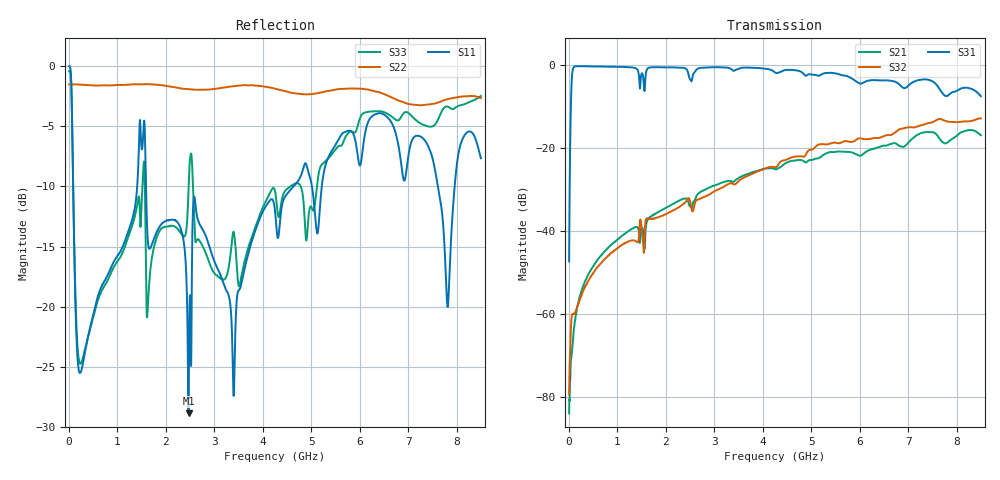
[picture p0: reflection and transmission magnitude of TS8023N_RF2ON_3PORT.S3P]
!Agilent Technologies,E5071C,MY46522130,B.12.04
!Date: Thu Jul 17 20:32:42 2025
!Data & Calibration Information:
!Freq	S11:SOLT3(ON)	S13:SOLT3(ON)	S14:SOLT3(ON)
!	S31:SOLT3(ON)	S33:SOLT3(ON)	S34:SOLT3(ON)
!	S41:SOLT3(ON)	S43:SOLT3(ON)	S44:SOLT3(ON)
!PortZ  Port1:50+j0  Port3:50+j0  Port4:50+j0
!Above PortZ is port z conversion or system Z0 setting when saving the data.
!When reading, reference impedance value at option line is always used.
# Hz S dB R 50
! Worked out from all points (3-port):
!   1601 points, 10 MHz to 8.5 GHz, reference 50 ohm
!   strongest paths, dB at 10 MHz, 2.132 GHz, 4.255 GHz, 6.378 GHz, 8.5 GHz:
!     S31: -47.3, -0.5, -1.7, -3.6, -7.4
!     S32: -79.4, -35.1, -24.6, -17.5, -12.8
!     S21: -84.0, -33.6, -25.1, -19.8, -16.8
!   lowest |S11| = -28.9 dB at 2.472 GHz (marker M1), VSWR 1.07, Z = 50.7 - j3.57 ohm
!   |S11| at or under -10 dB: 92.97 MHz to 1.413 GHz (1.32 GHz wide, 175 % of centre); 1.595 GHz to 4.636 GHz (3.041 GHz wide, 97.6 % of centre); 7.614 GHz to 7.959 GHz (345.3 MHz wide, 4.43 % of centre)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
1e7  0.00 163.0  -84.50 89.5  -47.36 -111.1
     -84.01 79.7  -1.52 179.8  -79.41 -109.2
     -47.31 -110.6  -79.43 -111.5  -0.42 162.0
6.836875e7  -3.80 42.9  -69.42 -74.2  -2.70 128.9
            -69.32 -74.2  -1.51 179.1  -60.24 137.2
            -2.71 128.8  -60.29 136.2  -3.84 35.4
1.267375e8  -17.56 -19.3  -61.94 169.8  -0.25 60.6
            -61.99 168.3  -1.51 178.4  -59.87 98.6
            -0.25 60.6  -60.00 100.3  -16.88 -35.9
4.238875e8  -22.10 -64.3  -50.08 112.0  -0.19 9.1
            -50.07 112.2  -1.57 174.4  -51.68 94.7
            -0.19 9.2  -51.68 94.4  -22.15 -87.6
1.522281e9  -6.65 -107.0  -39.21 94.0  -2.04 -28.2
            -39.23 93.9  -1.50 158.7  -40.78 83.4
            -2.04 -28.2  -40.76 83.3  -9.94 -145.2
2.4721e9  -28.86 -77.5  -33.23 82.3  -2.16 -54.7
          -33.16 82.5  -1.91 145.9  -32.03 86.0
          -2.16 -54.7  -32.07 86.0  -10.19 -125.0
4.255e9  -12.02 154.4  -25.17 66.8  -1.69 -83.5
         -25.06 67.2  -1.87 125.0  -24.46 73.9
         -1.70 -83.6  -24.58 73.5  -10.38 -167.3
6.478319e9  -3.96 142.5  -19.46 33.4  -3.62 -122.3
            -19.40 33.3  -2.27 97.0  -17.06 22.9
            -3.58 -122.3  -17.14 23.4  -3.78 154.3
7.815494e9  -20.02 131.9  -18.92 10.5  -7.31 -144.0
            -18.56 8.4  -2.74 56.1  -13.40 -14.8
            -7.30 -144.0  -13.56 -12.0  -3.36 116.6
8.5e9  -7.65 100.1  -16.77 -6.8  -7.45 -159.3
       -16.84 -5.3  -2.65 62.4  -12.74 -20.9
       -7.42 -159.1  -12.78 -22.1  -2.47 102.8
